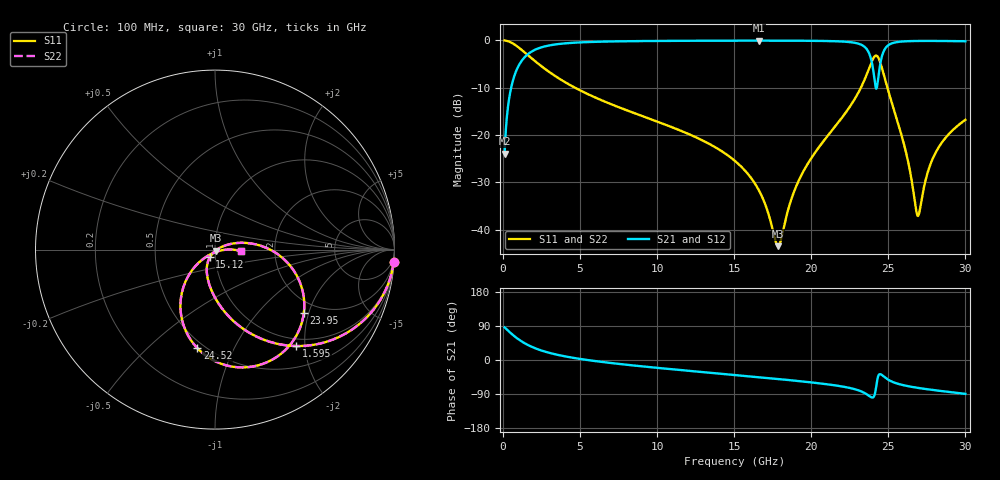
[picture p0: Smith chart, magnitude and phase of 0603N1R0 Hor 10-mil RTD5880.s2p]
# GHz S MA R 50
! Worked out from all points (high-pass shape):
!   3201 points, 100 MHz to 30 GHz, reference 50 ohm
!   highest |S21| = -0.06 dB at 16.63 GHz (marker M1); lowest = -24.0 dB at 100 MHz (marker M2)
!   |S21| within 3 dB of the highest: 1.56 GHz to 23.79 GHz (22.23 GHz wide, 175 % of centre); 24.61 GHz to end of sweep
!   lowest |S11| = -43.5 dB at 17.84 GHz (marker M3), VSWR 1.01, Z = 50.4 - j0.535 ohm
!   |S11| at or under -10 dB: 4.667 GHz to 23.22 GHz (18.55 GHz wide, 133 % of centre); 24.94 GHz to end of sweep
!   |S22| runs from -43.5 to 0.0 dB; largest |S21 - S12| = 0
!   S11 on the Smith chart (normalised r, x): 100 MHz: 1, -29; 1.595 GHz: 0.86, -1.82; 15.12 GHz: 0.94, -0.08; 23.95 GHz: 1.66, -1.86; 24.52 GHz: 0.46, -0.73; 30 GHz: 1.34, -0.02
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0.1  0.998 -3.9  0.06335 86.1  0.06335 86.1  0.998 -3.9
0.6139062  0.9316 -23.1  0.3631 66.9  0.3631 66.9  0.9316 -23.1
1.595  0.7019 -50.0  0.7112 40.0  0.7112 40.0  0.7019 -50.0
2.968531  0.4669 -70.5  0.8825 19.2  0.8825 19.2  0.4669 -70.5
5.089563  0.2915 -87.2  0.9539 2.2  0.9539 2.2  0.2915 -87.2
10.06978  0.1374 -109.3  0.9864 -21.0  0.9864 -21.0  0.1374 -109.3
15.05  0.0532 -123.8  0.993 -39.6  0.993 -39.6  0.0532 -123.8
15.11541  0.0521 -123.9  0.993 -39.9  0.993 -39.9  0.0521 -123.9
16.62909  0.02553 -121.8  0.9934 -45.5  0.9934 -45.5  0.02553 -121.8
17.84378  0.006697 -52.4  0.9931 -50.2  0.9931 -50.2  0.006697 -52.4
18.89963  0.02567 18.7  0.992 -54.4  0.992 -54.4  0.02567 18.7
20.03956  0.05825 22.1  0.9893 -59.3  0.9893 -59.3  0.05825 22.1
23.09497  0.2888 1.7  0.9189 -80.5  0.9189 -80.5  0.2888 1.7
23.59019  0.4337 -12.7  0.8118 -90.2  0.8118 -90.2  0.4337 -12.7
23.94525  0.6077 -35.5  0.568 -99.1  0.568 -99.1  0.6077 -35.5
24.22556  0.6906 -67.0  0.3091 -66.3  0.3091 -66.3  0.6906 -67.0
24.51522  0.5574 -100.2  0.6102 -37.9  0.6102 -37.9  0.5574 -100.2
25.01978  0.2847 -129.1  0.8938 -52.7  0.8938 -52.7  0.2847 -129.1
26.12234  0.06808 -141.2  0.978 -67.8  0.978 -67.8  0.06808 -141.2
26.91656  0.01397 -70.9  0.9857 -73.6  0.9857 -73.6  0.01397 -70.9
28.04716  0.06415 -0.2  0.9862 -79.9  0.9862 -79.9  0.06415 -0.2
30  0.1447 -3.5  0.9787 -89.3  0.9787 -89.3  0.1447 -3.5
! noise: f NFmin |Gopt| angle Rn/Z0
0.1  0.0004809  0.9566  1.324  0.002498
3.417  0.004051  0.811  10.47  0.004432
6.743  0.006799  0.7822  19.84  0.006219
10.06  0.009325  0.767  29.13  0.007638
13.39  0.01187  0.76  38.28  0.008962
16.7  0.0147  0.7613  47.19  0.01053
20.03  0.01913  0.7809  55.87  0.01403
23.35  0.05535  0.9069  64.44  0.0935
26.67  0.0286  0.8078  72.94  0.02016
30  0.02524  0.7645  80.74  0.0128
